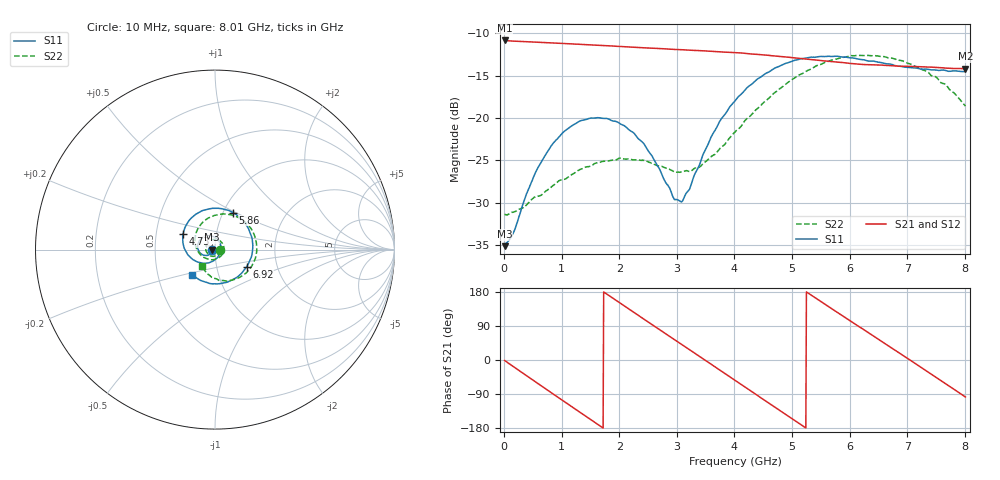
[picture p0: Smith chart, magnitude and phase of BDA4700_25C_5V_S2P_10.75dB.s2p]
!Agilent Technologies,E5071B,MY42404982,A.09.10
!Date: Mon Oct 20 13:31:27 2025
!Data & Calibration Information:
!Freq	S11:SOLT2(ON)	S21:SOLT2(ON)	S12:SOLT2(ON)	S22:SOLT2(ON)
# Hz S RI R 50
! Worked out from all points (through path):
!   801 points, 10 MHz to 8.01 GHz, reference 50 ohm
!   highest |S21| = -10.86 dB at 10 MHz (marker M1); lowest = -14.2 dB at 8.01 GHz (marker M2)
!   group delay of S21, straight-line fit = 283 ps
!   lowest |S11| = -35.1 dB at 10 MHz (marker M3), VSWR 1.04, Z = 48.3 - j0.112 ohm
!   |S11| at or under -10 dB: start of sweep to end of sweep
!   |S22| runs from -31.5 to -12.6 dB; largest |S21 - S12| = 0.0022
!   S11 on the Smith chart (normalised r, x): 10 MHz: 0.97, -0.00; 4.73 GHz: 0.69, +0.13; 5.86 GHz: 1.11, +0.48; 6.92 GHz: 1.39, -0.28; 8.01 GHz: 0.75, -0.22
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1e7  -0.0175 -0.00116  0.2863 -0.00632  0.2861 -0.0065  0.0271 -0.0014
1.6e8  -0.0185 -0.00967  0.2711 -0.0838  0.2711 -0.0839  0.0264 -0.0088
3.3e8  -0.0239 -0.0199  0.2308 -0.1621  0.2307 -0.1624  0.0223 -0.0192
7.2e8  -0.0508 -0.0328  0.0679 -0.2696  0.0681 -0.2697  -0.00114 -0.0368
1.02e9  -0.0785 -0.0227  -0.0803 -0.2629  -0.0805 -0.263  -0.0276 -0.0333
1.35e9  -0.0964 0.00808  -0.2115 -0.17  -0.2116 -0.1702  -0.0495 -0.00688
1.93e9  -0.0656 0.0694  -0.2472 0.0952  -0.2472 0.0953  -0.0263 0.0498
2.32e9  -0.0163 0.0743  -0.1262 0.2279  -0.1261 0.2279  0.0174 0.0537
2.68e9  0.0223 0.046  0.0348 0.2543  0.0347 0.2543  0.0466 0.0233
2.95e9  0.0323 0.00828  0.1468 0.2069  0.1467 0.2067  0.0475 -0.0081
3.09e9  0.0296 -0.0125  0.1926 0.1633  0.1918 0.1638  0.041 -0.0246
3.54e9  -0.0181 -0.0671  0.2467 -0.0238  0.2467 -0.0241  -0.00795 -0.0561
4.01e9  -0.1088 -0.0635  0.144 -0.1952  0.1442 -0.195  -0.075 -0.0342
4.37e9  -0.1663 -0.00349  -0.00162 -0.2373  -0.00196 -0.2377  -0.1091 0.0227
4.73e9  -0.178 0.088  -0.1405 -0.1839  -0.14 -0.1844  -0.1027 0.0997
5.35e9  -0.0618 0.2196  -0.2171 0.0402  -0.2174 0.0396  0.0205 0.1945
5.86e9  0.0986 0.2065  -0.1003 0.1871  -0.1002 0.1871  0.164 0.157
6.27e9  0.1894 0.1105  0.0435 0.2017  0.0454 0.201  0.2286 0.0476
6.68e9  0.2064 -0.0245  0.1632 0.1214  0.1636 0.1212  0.2138 -0.0729
6.92e9  0.176 -0.0962  0.1967 0.0449  0.1966 0.044  0.1735 -0.1301
7.47e9  0.0286 -0.1896  0.1461 -0.1349  0.1457 -0.1353  0.0303 -0.1731
8.01e9  -0.1263 -0.1395  -0.0258 -0.1932  -0.0256 -0.1934  -0.0711 -0.0933
